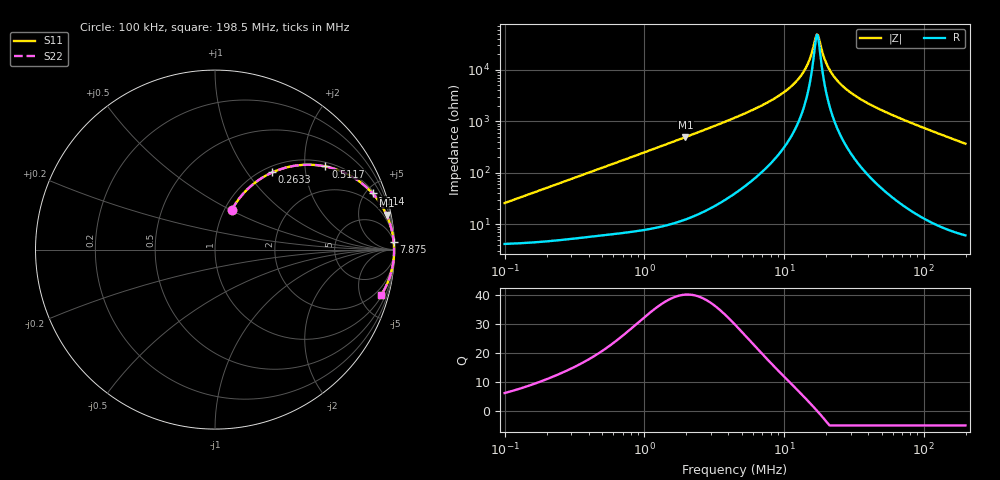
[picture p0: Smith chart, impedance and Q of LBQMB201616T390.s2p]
! LBQMB201616T390  S-PARAMETER MODEL  ( General Type )
! Model Generated by TAIYO YUDEN Corporation (http://www.ty-top.com)
! Version 1.0
! TAIYO YUDEN Control No. 191025NI43SB-FBB
! Copyright(c) 2019 TAIYO YUDEN CO.,LTD. All Rights Reserved.
! Product Description (link to TY-COMPAS)
! https://ds.yuden.co.jp/TYCOMPAS/or/detail?pn=LBQMB201616T390J&u=M
! Products Name : Inductors
! Characteristics :
!  Inductance : 39 uH , SRF(min) : 14 MHz , DC Resistance(max) : 5.07 Ohm , Rated Current : 120 mA
!  Case Size : 2.0 x 1.6 / 0.079 x 0.063 [mm/inch] , Thickness : 1.6 / 0.063 [mm/inch]
!  (Conditions: Temperature = 25 degC , DC Bias Current/Voltage = 0A / 0V)
! External Node Assignments :
!  1  o---GGG---o  2
! GND o---------o GND
! Frequency Range : 0.1MHz  -  198.534594MHz  [ 402 STEP ]
# MHz S RI R 50
! Freq[MHz].  S11 Real  S11 Imag  S21 Real  S21 Imag  S12 Real  S12 Imag  S22 Real  S22 Imag
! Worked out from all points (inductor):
!   401 points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, 100 kHz to 198.5 MHz, reference 50 ohm
!   read as one part in series: L = 40.4 uH near 103.9 kHz
!   highest Q = 40 at 1.97 MHz (marker M1), where L = 39.9 uH
!   self-resonance near 17.15 MHz
!   S11 on the Smith chart (normalised r, x): 100 kHz: 1.08, +0.51; 263.3 kHz: 1.10, +1.33; 511.7 kHz: 1.12, +2.56; 1.114 MHz: 1.16, +5.54; 7.875 MHz: 4, +49; 198.5 MHz: 1.12, -7.34
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0.1  0.0936 0.2212  0.9064 -0.2212  0.9064 -0.2212  0.0936 0.2212
0.166957  0.1774 0.333  0.8226 -0.333  0.8226 -0.333  0.1774 0.333
0.263314  0.3192 0.4302  0.6808 -0.4302  0.6808 -0.4302  0.3192 0.4302
0.356769  0.4487 0.4679  0.5513 -0.4679  0.5513 -0.4679  0.4487 0.4679
0.511723  0.6153 0.4633  0.3847 -0.4633  0.3847 -0.4633  0.6153 0.4633
1.114456  0.8779 0.3131  0.1221 -0.3131  0.1221 -0.3131  0.8779 0.3131
1.272844  0.9031 0.2823  0.0969 -0.2823  0.0969 -0.2823  0.9031 0.2823
1.969703  0.9561 0.1927  0.0439 -0.1927  0.0439 -0.1927  0.9561 0.1927
4.541117  0.9904 0.082  0.00961 -0.082  0.00961 -0.082  0.9904 0.082
7.875095  0.996 0.0405  0.00405 -0.0405  0.00405 -0.0405  0.996 0.0405
10.46947  0.9972 0.0244  0.00285 -0.0244  0.00285 -0.0244  0.9972 0.0244
12.65816  0.9976 0.0148  0.00238 -0.0148  0.00238 -0.0148  0.9976 0.0148
14.45715  0.9978 0.00837  0.00217 -0.00837  0.00217 -0.00837  0.9978 0.00837
15.89665  0.9979 0.00387  0.00207 -0.00387  0.00207 -0.00387  0.9979 0.00387
16.82827  0.998 0.00119  0.00203 -0.00119  0.00203 -0.00119  0.998 0.00119
17.47948  0.998 -0.0006  0.00201 0.0006  0.00201 0.0006  0.998 -0.0006
20.3463  0.998 -0.0078  0.00201 0.0078  0.00201 0.0078  0.998 -0.0078
21.95147  0.9979 -0.0115  0.00205 0.0115  0.00205 0.0115  0.9979 -0.0115
24.59978  0.9978 -0.0171  0.00217 0.0171  0.00217 0.0171  0.9978 -0.0171
33.96951  0.997 -0.0345  0.00301 0.0345  0.00301 0.0345  0.997 -0.0345
56.71438  0.9932 -0.0704  0.00685 0.0704  0.00685 0.0704  0.9932 -0.0704
198.5346  0.9274 -0.2514  0.0726 0.2514  0.0726 0.2514  0.9274 -0.2514
